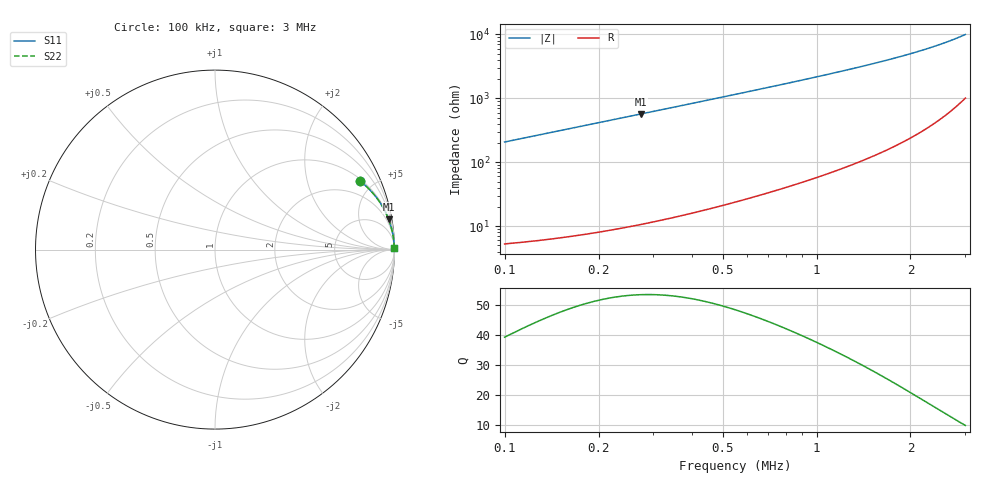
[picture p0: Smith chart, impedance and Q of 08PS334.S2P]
! Coilcraft 0805PS-334 Power Chip Inductor
! 5 February 2003
# MHZ S MA R 50
!Freq  MagS11  AngS11  MagS21  AngS21  MagS12  AngS12  MagS22  AngS22
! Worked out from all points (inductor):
!   402 points, 100 kHz to 3 MHz, reference 50 ohm
!   read as one part in series: L = 330 uH near 114.5 kHz
!   highest Q = 53.5 at 273.6 kHz (marker M1), where L = 331 uH
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0.1  0.892 25.5  0.4299 -63.1  0.4299 -63.1  0.892 25.5
0.114464  0.9139 22.6  0.3848 -66.0  0.3848 -66.0  0.9139 22.6
0.13616  0.9363 19.3  0.3313 -69.4  0.3313 -69.4  0.9363 19.3
0.150624  0.9467 17.6  0.3028 -71.2  0.3028 -71.2  0.9467 17.6
0.17232  0.9581 15.5  0.2678 -73.3  0.2678 -73.3  0.9581 15.5
0.194016  0.9662 13.9  0.2398 -75.0  0.2398 -75.0  0.9662 13.9
0.222944  0.9737 12.1  0.2102 -76.8  0.2102 -76.8  0.9737 12.1
0.273568  0.9818 9.9  0.1725 -79.0  0.1725 -79.0  0.9818 9.9
0.338656  0.9875 8.0  0.14 -80.9  0.14 -80.9  0.9875 8.0
0.410976  0.9911 6.6  0.1155 -82.3  0.1155 -82.3  0.9911 6.6
0.490528  0.9934 5.5  0.09668 -83.3  0.09668 -83.3  0.9934 5.5
0.584544  0.995 4.6  0.08092 -84.2  0.08092 -84.2  0.995 4.6
0.685792  0.9961 3.9  0.06867 -84.8  0.06867 -84.8  0.9961 3.9
0.801504  0.9969 3.3  0.05837 -85.3  0.05837 -85.3  0.9969 3.3
0.93168  0.9975 2.9  0.04975 -85.7  0.04975 -85.7  0.9975 2.9
1.069088  0.9979 2.5  0.04285 -86.0  0.04285 -86.0  0.9979 2.5
1.29328  0.9983 2.0  0.03461 -86.2  0.03461 -86.2  0.9983 2.0
1.553632  0.9986 1.6  0.02785 -86.3  0.02785 -86.3  0.9986 1.6
1.777824  0.9987 1.3  0.02349 -86.3  0.02349 -86.3  0.9987 1.3
2.038176  0.9989 1.1  0.01951 -86.1  0.01951 -86.1  0.9989 1.1
2.52272  0.9989 0.8  0.014 -85.2  0.014 -85.2  0.9989 0.8
3  0.9989 0.6  0.01001 -83.6  0.01001 -83.6  0.9989 0.6
